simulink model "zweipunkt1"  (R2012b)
settings: Solver=ode45  StartTime=0.0  StopTime=10.0  RelTol=1e-3
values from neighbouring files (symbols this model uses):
  hy = 0.01    [fuellstnd_3.m]    (also in fuellstnd_31.m; regulator_1.m = 2; zweipunkt_1.m = 20; zweipunkt_2.m = 0)
  Kp = 10    [zweipunkt_1.m]    (also in zweipunkt_2.m; zweipunkt_21.m; zweipunkt_31.m; zweipunkt_32.m = 1)
  Tp = 1    [fuellstnd_2.m]    (also in fuellstnd_21.m = 0.1; fuellstnd_3.m = 0.1; fuellstnd_31.m = 0.01; regulator_1.m = 5)
  ysoll = y.signals.values(:,2)    [ohne_kalman_1.m]    (also in zweipunkt_1.m = 500; zweipunkt_2.m = 500; zweipunkt_21.m = 500; zweipunkt_31.m = 500)

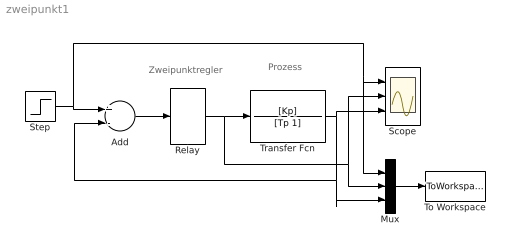
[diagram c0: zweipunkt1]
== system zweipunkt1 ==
  note: Zweipunktregler
  note: Prozess
  Add : Sum  Inputs=+-
  Mux : Mux  Inputs=3
  Relay : Relay  OnSwitchValue=hy  OffSwitchValue=-hy  OnOutputValue=Ustell  ZeroCross=off
  Scope : Scope  NumInputPorts=3
  Step : Step  Time=10  After=ysoll  SampleTime=0
  To Workspace : ToWorkspace  VariableName=y  SampleTime=-1  SaveFormat=Structure With Time
  Transfer Fcn : TransferFcn  Numerator=[Kp]  Denominator=[Tp 1]
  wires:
  Add/1 -> Relay/1
  Transfer Fcn/1 -> Scope/3, Mux/3, Add/2
  Step/1 -> Mux/1, Scope/1, Add/1
  Relay/1 -> Scope/2, Mux/2, Transfer Fcn/1
  Mux/1 -> To Workspace/1
